[IBIS Ver]   4.1
[File Name]   f771973xpt.ibs
[File Rev]   1.1
[Date]   DEC 06, 2019
[Source]   File originated at Texas Instruments
[Copyright]   (c) 2012, Texas Instruments Inc.
[Component]   f771973xpt
[Manufacturer] Texas Instruments
[Package]
| Variable   Typ   Min   Max
R_pkg   0.227   0.120   0.292
L_pkg   2.69E-9   1.93E-09   3.45E-09
C_pkg   2.74E-13   2.20E-13   4.26E-13
[Pin]	signal_name	model_name	R_pin	L_pin	C_pin
1	GPIO29	BCPF335585DSHYPBFZ	0.25941	3.0919E-09	2.4351E-13
2	GPIO28	BCF3385DSHYPBFZ_USF	0.23606	2.7405E-09	2.7713E-13
3	XRSN	BQ0491FS_USF	0.22061	2.5663E-09	2.5848E-13
4	A6	ICF33SHYPB_USF	0.28245	3.2561E-09	3.2289E-13
5	A3	ICF33SHYPB_USF	0.26646	3.0106E-09	2.9004E-13
6	A2	ICF33SHYPB_USF	0.24645	2.8148E-09	2.6028E-13
7	A15	ICF33SHYPB_USF	0.23123	2.6138E-09	2.4369E-13
8	A11	ICF33SHYPB_USF	0.22264	2.5157E-09	2.4792E-13
9	A5	ICF33SHYPB_USF	0.2176	2.4751E-09	2.5748E-13
10	A1	ICF33SHYPB_USF	0.221	2.5269E-09	2.6653E-13
11   A0	ICF33SHYPB_USF	0.23693	2.6747E-09	2.8201E-13
12	VREFHIAC	NC	0.13814	2.299E-09	2.844E-13
13	VREFLOAC	NC	0.13637	2.3105E-09	2.7964E-13
14	A12	ICF33SHYPB_USF	0.22612	2.5696E-09	2.801E-13
15	A7	ICF33SHYPB_USF	0.21108	2.4082E-09	2.6154E-13
16	A8	ICF33SHYPB_USF	0.20949	2.3462E-09	2.5429E-13
17	VSSA	NC	0.12003	1.9347E-09	2.8874E-13
18	VDDA	NC	0.12462	2.0226E-09	2.8835E-13
19	A4	ICF33SHYPB_USF	0.23926	2.6395E-09	2.5833E-13
20	C8	ICF33SHYPB_USF	0.25542	2.8708E-09	2.7685E-13
21	A10	ICF33SHYPB_USF	0.27986	3.1631E-09	2.8865E-13
22	VSS	NC	0.25716	2.9826E-09	2.6508E-13
23	GPIO13	BCF3385DSHYPBFZ_USF	0.24694	2.874E-09	2.7658E-13
24	GPIO12	BCF3385DSHYPBFZ_USF	0.27087	3.1672E-09	2.5224E-13
25	GPIO33	BCPF335585DSHYPBFZ	0.24318	2.8761E-09	2.3782E-13
26	GPIO16	BCF3385DSHYPBFZ_USF	0.22624	2.6468E-09	2.6309E-13
27	GPIO24	BCPF335585DSHYPBFZ	0.22475	2.6089E-09	2.528E-13
28	TCK	BCF3355DSHYPBFZ_TMS_USF	0.21946	2.5235E-09	2.4928E-13
29	TDO_GPIO37	BCPF335585DSHYPBFZ	0.22358	2.5342E-09	2.5036E-13
30	TMS	BCF3355DSHYPBFZ_TMS_USF	0.22142	2.5275E-09	2.4265E-13
31	TDI_GPIO35	BCF3385DSHYPBFZ_USF	0.2324	2.6413E-09	2.4841E-13
32	GPIO32	BCPF335585DSHYPBFZ	0.25413	2.858E-09	2.7843E-13
33	GPIO18_X2	BCPF335585DSHYPBFZ	0.2705	3.0961E-09	3.5245E-13
34	GPIO19_X1	BCF3385DSHYPBFZ_USF	0.28192	3.2035E-09	3.7023E-13
35	VDDSFL	NC	0.16955	2.9214E-09	4.2675E-13
36	VDD	NC	0.29198	3.4219E-09	3.8604E-13
37	VSS	NC	0.29231	3.4515E-09	2.9642E-13
38	GPIO4	BCF3385DSHYPBFZ_USF	0.21567	2.5508E-09	2.5641E-13
39	GPIO3	BCF3385DSHYPBFZ_USF	0.21158	2.4648E-09	2.5362E-13
40	GPIO2	BCF3385DSHYPBFZ_USF	0.20478	2.3668E-09	2.4662E-13
41	GPIO1	BCPF335585DSHYPBFZ	0.21473	2.4416E-09	2.4208E-13
42	GPIO0	BCF3385DSHYPBFZ_USF	0.21637	2.4612E-09	2.278E-13
43	GPIO7	BCF3385DSHYPBFZ_USF	0.20959	2.4021E-09	2.204E-13
44	VSS	NC	0.2153	2.4686E-09	2.4702E-13
45	VDD	NC	0.23483	2.6923E-09	3.26E-13
46	VDDSFL	NC	0.21857	2.6156E-09	3.0232E-13
47	GPIO5	BCF3385DSHYPBFZ_USF	0.23867	2.8188E-09	2.7315E-13
48	GPIO6	BCF3385DSHYPBFZ_USF	0.2323	2.7652E-09	2.2867E-13
| End of package information
|   Component IQ0440FS_VREGENZ_USF
[Component]   IQ0440FS_VREGENZ_USF
[Manufacturer]   Texas Instruments
[Package]
|  variable   typ   min   max
R_pkg   0   0   0
L_pkg   0   0   0
C_pkg   0   0   0
[Pin]   signal_name   model_name   R_pin   L_pin   C_pin
VSS   VSS   GND
VDDS   VDDS   POWER
PAD   PAD   IQ0440FS_VREGENZ_USF
[Model Selector] IQ0440FS_VREGENZ_USF
VREGENZ_WK_PD_ON_3P3  Cell operated at 3.3(nom)
|VREGENZ_WK_PD_ON_3P3; WEAK_PULLDOWN_ON
VREGENZ_WK_PD_OFF_3P3  Cell operated at 3.3(nom)
|   Component ICF33SHYPB_USF
[Component]   ICF33SHYPB_USF
[Manufacturer]   Texas Instruments
[Package]
|  variable   typ   min   max
R_pkg   0   0   0
L_pkg   0   0   0
C_pkg   0   0   0
[Pin]   signal_name   model_name   R_pin   L_pin   C_pin
VSS   VSS   GND
VDDS   VDDS   POWER
PAD   PAD   ICF33SHYPB_USF
[Model Selector] ICF33SHYPB_USF
ICF_WK_PUPD_OFF_3P3  Cell operated at 3.3(nom)
|ICF_WK_PUPD_OFF_3P3; WEAK_PULL_OFF
ICF_WK_PU_ON_3P3  Cell operated at 3.3(nom)
|ICF_WK_PU_ON_3P3; WEAK_PULLUP_ON
ICF_WK_PD_ON_3P3  Cell operated at 3.3(nom)
|   Component ICF33SHYPB_FS_SFII_CUS
[Component]   ICF33SHYPB_FS_SFII_CUS
[Manufacturer]   Texas Instruments
[Package]
|  variable   typ   min   max
R_pkg   0   0   0
L_pkg   0   0   0
C_pkg   0   0   0
[Pin]   signal_name   model_name   R_pin   L_pin   C_pin
VSS   VSS   GND
VDDS   VDDS   POWER
PAD   PAD   ICF33SHYPB_FS_SFII_CUS
[Model Selector] ICF33SHYPB_FS_SFII_CUS
CUS_WK_PUPD_OFF_3P3  Cell operated at 3.3(nom)
|CUS_WK_PUPD_OFF_3P3; WEAK_PULL_OFF
CUS_WK_PU_ON_3P3  Cell operated at 3.3(nom)
|CUS_WK_PU_ON_3P3; WEAK_PULLUP_ON
CUS_WK_PD_ON_3P3  Cell operated at 3.3(nom)
|   Component BT3308BT5FSHYPB_SFII
[Component]   BT3308BT5FSHYPB_SFII
[Manufacturer]   Texas Instruments
[Package]
|  variable   typ   min   max
R_pkg   0   0   0
L_pkg   0   0   0
C_pkg   0   0   0
[Pin]   signal_name   model_name   R_pin   L_pin   C_pin
VSS   VSS   GND
VDDS   VDDS   POWER
PAD   PAD   BT3308BT5FSHYPB_SFII
[Model Selector] BT3308BT5FSHYPB_SFII
BT_OPEN_DRAIN_6MA_3P3  Cell operated at 3.3(nom)
|BT_OPEN_DRAIN_6MA_3P3
BT_WEAK_PD_ON_3P3  Cell operated at 3.3(nom)
|BT_WEAK_PD_ON_3P3
BT_OPEN_DRAIN_3MA_3P3  Cell operated at 3.3(nom)
|BT_OPEN_DRAIN_3MA_3P3
BT_DRIVER_MODE_6MA_3P3  Cell operated at 3.3(nom)
|BT_DRIVER_MODE_6MA_3P3
BT_DRIVER_MODE_3MA_3P3  Cell operated at 3.3(nom)
|BT_DRIVER_MODE_3MA_3P3
BT_WEAK_PU_ON_3P3  Cell operated at 3.3(nom)
|   Component BQ0491FS_USF
[Component]   BQ0491FS_USF
[Manufacturer]   Texas Instruments
[Package]
|  variable   typ   min   max
R_pkg   0   0   0
L_pkg   0   0   0
C_pkg   0   0   0
[Pin]   signal_name   model_name   R_pin   L_pin   C_pin
VSS   VSS   GND
VDDS   VDDS   POWER
PAD   PAD   BQ0491FS_USF
[Model Selector] BQ0491FS_USF
XRSN_WK_PU_ON_3P3  Cell operated at 3.3(nom)
|XRSN_WK_PU_ON_3P3; WEAK_PULLUP_ON
XRSN_OPEN_DRAIN  Cell operated at 3.3(nom)
|   Component BCPF335585DSHYPBFZ
[Component]   BCPF335585DSHYPBFZ
[Manufacturer]   Texas Instruments
[Package]
|  variable   typ   min   max
R_pkg   0   0   0
L_pkg   0   0   0
C_pkg   0   0   0
[Pin]   signal_name   model_name   R_pin   L_pin   C_pin
VSS   VSS   GND
VDDS   VDDS   POWER
PAD   PAD   BCPF335585DSHYPBFZ
[Model Selector] BCPF335585DSHYPBFZ
BCPF_WK_PU_ON_3P3  Cell operated at 3.3(nom)
|BCPF_WK_PU_ON_3P3; WEAK_PULLUP_ON
BCPF_DRIVER_4MA_3P3  Cell operated at 3.3(nom)
|BCPF_DRIVER_4MA_3P3
BCPF_DRIVER_2MA_3P3  Cell operated at 3.3(nom)
|BCPF_DRIVER_2MA_3P3
BCPF_WK_PD_ON_3P3  Cell operated at 3.3(nom)
|   Component BCF3385DSHYPBFZ_USF
[Component]   BCF3385DSHYPBFZ_USF
[Manufacturer]   Texas Instruments
[Package]
|  variable   typ   min   max
R_pkg   0   0   0
L_pkg   0   0   0
C_pkg   0   0   0
[Pin]   signal_name   model_name   R_pin   L_pin   C_pin
VSS   VSS   GND
VDDS   VDDS   POWER
PAD   PAD   BCF3385DSHYPBFZ_USF
[Model Selector] BCF3385DSHYPBFZ_USF
BCF3385DUSF_WK_PU  Cell operated at 3.3(nom)
| BCF3385DUSF_WK_PU; WEAK_PULLUP_ON
BCF3385DUSF_DRIVER_3P3  Cell operated at 3.3(nom)
|BCF3385DUSF_DRIVER_3P3
BCF3385DUSF_WK_PD  Cell operated at 3.3(nom)
|   Component BCF3385DSHYPBFZ
[Component]   BCF3385DSHYPBFZ
[Manufacturer]   Texas Instruments
[Package]
|  variable   typ   min   max
R_pkg   0   0   0
L_pkg   0   0   0
C_pkg   0   0   0
[Pin]   signal_name   model_name   R_pin   L_pin   C_pin
VSS   VSS   GND
VDDS   VDDS   POWER
PAD   PAD   BCF3385DSHYPBFZ
[Model Selector] BCF3385DSHYPBFZ
BCF3385D_WK_PU_3P3  Cell operated at 3.3(nom)
|BCF3385D_WK_PU_3P3; WEAK_PULLUP_ON
BCF3385D_DRIVER_3P3  Cell operated at 3.3(nom)
|BCF3385D_DRIVER_3P3
BCF3385D_WK_PD_3P3  Cell operated at 3.3(nom)
|   Component BCF3355DSHYPBFZ_TMS_USF
[Component]   BCF3355DSHYPBFZ_TMS_USF
[Manufacturer]   Texas Instruments
[Package]
|  variable   typ   min   max
R_pkg   0   0   0
L_pkg   0   0   0
C_pkg   0   0   0
[Pin]   signal_name   model_name   R_pin   L_pin   C_pin
VSS   VSS   GND
VDDS   VDDS   POWER
PAD   PAD   BCF3355DSHYPBFZ_TMS_USF
[Model Selector] BCF3355DSHYPBFZ_TMS_USF
TMS_WK_PU_ON_3P3  Cell operated at 3.3(nom)
|TMS_WK_PU_ON_3P3; WEAK_PULLUP_ON
TMS_DRIVER_3P3  Cell operated at 3.3(nom)
|TMS_DRIVER_3P3
TMS_WK_PD_ON_3P3  Cell operated at 3.3(nom)
|   Component BCF3335DSHYPBFZ
[Component]   BCF3335DSHYPBFZ
[Manufacturer]   Texas Instruments
[Package]
|  variable   typ   min   max
R_pkg   0   0   0
L_pkg   0   0   0
C_pkg   0   0   0
[Pin]   signal_name   model_name   R_pin   L_pin   C_pin
VSS   VSS   GND
VDDS   VDDS   POWER
PAD   PAD   BCF3335DSHYPBFZ
[Model Selector] BCF3335DSHYPBFZ
BCF3335D_WK_PU_3P3  Cell operated at 3.3(nom)
|BCF3335D_WK_PU_3P3; WEAK_PULLUP_ON
BCF3335D_DRIVER_3P3  Cell operated at 3.3(nom)
|BCF3335D_DRIVER_3P3
BCF3335D_WK_PD_3P3  Cell operated at 3.3(nom)
| Models and submodels in the file (32): VREGENZ_WK_PD_ON_3P3 (Input), VREGENZ_WK_PD_OFF_3P3 (Input), ICF_WK_PUPD_OFF_3P3 (Input), ICF_WK_PU_ON_3P3 (Input), ICF_WK_PD_ON_3P3 (Input), CUS_WK_PUPD_OFF_3P3 (Input), CUS_WK_PU_ON_3P3 (Input), CUS_WK_PD_ON_3P3 (Input), BT_OPEN_DRAIN_6MA_3P3 (I/O_open_drain), BT_WEAK_PD_ON_3P3 (Input), BT_OPEN_DRAIN_3MA_3P3 (I/O_open_drain), BT_DRIVER_MODE_6MA_3P3 (I/O), BT_DRIVER_MODE_3MA_3P3 (I/O), BT_WEAK_PU_ON_3P3 (Input), XRSN_WK_PU_ON_3P3 (Input), XRSN_OPEN_DRAIN (I/O_open_drain), BCPF_WK_PU_ON_3P3 (Input), BCPF_DRIVER_4MA_3P3 (I/O), BCPF_DRIVER_2MA_3P3 (I/O), BCPF_WK_PD_ON_3P3 (Input), BCF3385DUSF_WK_PU (Input), BCF3385DUSF_DRIVER_3P3 (I/O), BCF3385DUSF_WK_PD (Input), BCF3385D_WK_PU_3P3 (Input), BCF3385D_DRIVER_3P3 (I/O), BCF3385D_WK_PD_3P3 (Input), TMS_WK_PU_ON_3P3 (Input), TMS_DRIVER_3P3 (I/O), TMS_WK_PD_ON_3P3 (Input), BCF3335D_WK_PU_3P3 (Input), BCF3335D_DRIVER_3P3 (I/O), BCF3335D_WK_PD_3P3 (Input)
